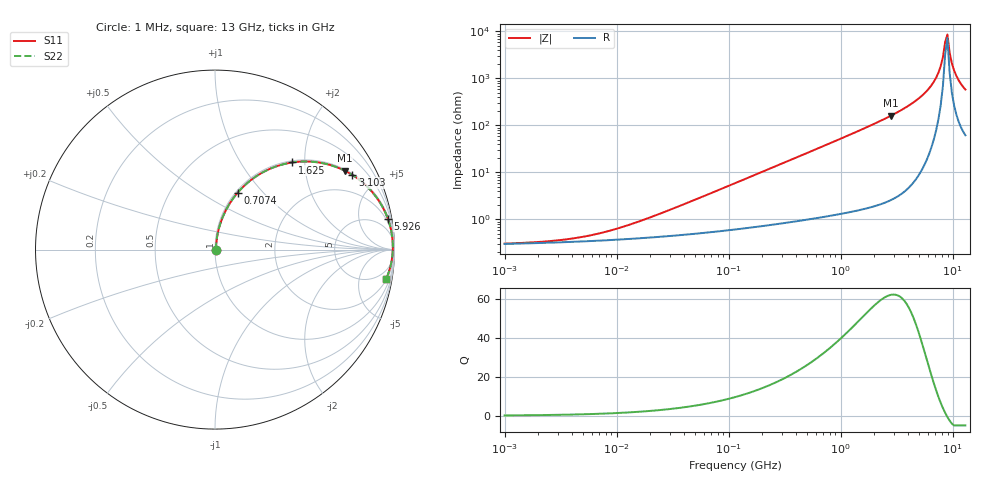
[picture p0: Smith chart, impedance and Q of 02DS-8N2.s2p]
# MHz S MA R 50
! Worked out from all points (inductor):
!   206 points, 1 MHz to 13 GHz, reference 50 ohm
!   read as one part in series: L = 8.2 nH near 25.4 MHz
!   highest Q = 62.4 at 2.829 GHz (marker M1), where L = 9.13 nH
!   self-resonance near 8.577 GHz
!   S11 on the Smith chart (normalised r, x): 1 MHz: 1.01, +0.00; 707.4 MHz: 1.02, +0.73; 1.625 GHz: 1.03, +1.73; 3.103 GHz: 1.06, +3.65; 5.926 GHz: 1, +11; 13 GHz: 2, -12
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1  0.003054 9.7  0.997 -0.0  0.997 -0.0  0.003054 9.7
5.03942  0.004278 37.1  0.9966 -0.1  0.9966 -0.1  0.004278 37.1
10.0786  0.006362 54.1  0.9963 -0.3  0.9963 -0.3  0.006362 54.1
24.249  0.01315 70.4  0.9957 -0.7  0.9957 -0.7  0.01315 70.4
116.682  0.05997 80.7  0.9921 -3.4  0.9921 -3.4  0.05997 80.7
561.459  0.2765 71.9  0.9512 -16.0  0.9512 -16.0  0.2765 71.9
707.389  0.3411 68.3  0.9295 -19.9  0.9295 -19.9  0.3411 68.3
1625.11  0.6488 48.5  0.7486 -40.4  0.7486 -40.4  0.6488 48.5
2701.66  0.8318 32.8  0.5419 -56.3  0.5419 -56.3  0.8318 32.8
2829.43  0.8455 31.4  0.5207 -57.7  0.5207 -57.7  0.8455 31.4
3103.38  0.8709 28.5  0.4777 -60.6  0.4777 -60.6  0.8709 28.5
4491.37  0.9467 17.7  0.3038 -71.2  0.3038 -71.2  0.9467 17.7
5926.35  0.978 10.2  0.1769 -77.8  0.1769 -77.8  0.978 10.2
6807.55  0.9864 6.6  0.1152 -80.0  0.1152 -80.0  0.9864 6.6
7466.67  0.9896 4.3  0.0747 -79.9  0.0747 -79.9  0.9896 4.3
8189.61  0.9909 1.9  0.03503 -73.9  0.03503 -73.9  0.9909 1.9
8576.92  0.9908 0.8  0.01661 -56.0  0.01661 -56.0  0.9908 0.8
8982.54  0.9903 -0.4  0.0115 31.9  0.0115 31.9  0.9903 -0.4
9407.35  0.9892 -1.5  0.02815 66.8  0.02815 66.8  0.9892 -1.5
10318.2  0.9857 -3.8  0.06723 75.9  0.06723 75.9  0.9857 -3.8
11317.2  0.9803 -6.1  0.1071 76.3  0.1071 76.3  0.9803 -6.1
13000  0.9682 -9.6  0.1673 74.3  0.1673 74.3  0.9682 -9.6
